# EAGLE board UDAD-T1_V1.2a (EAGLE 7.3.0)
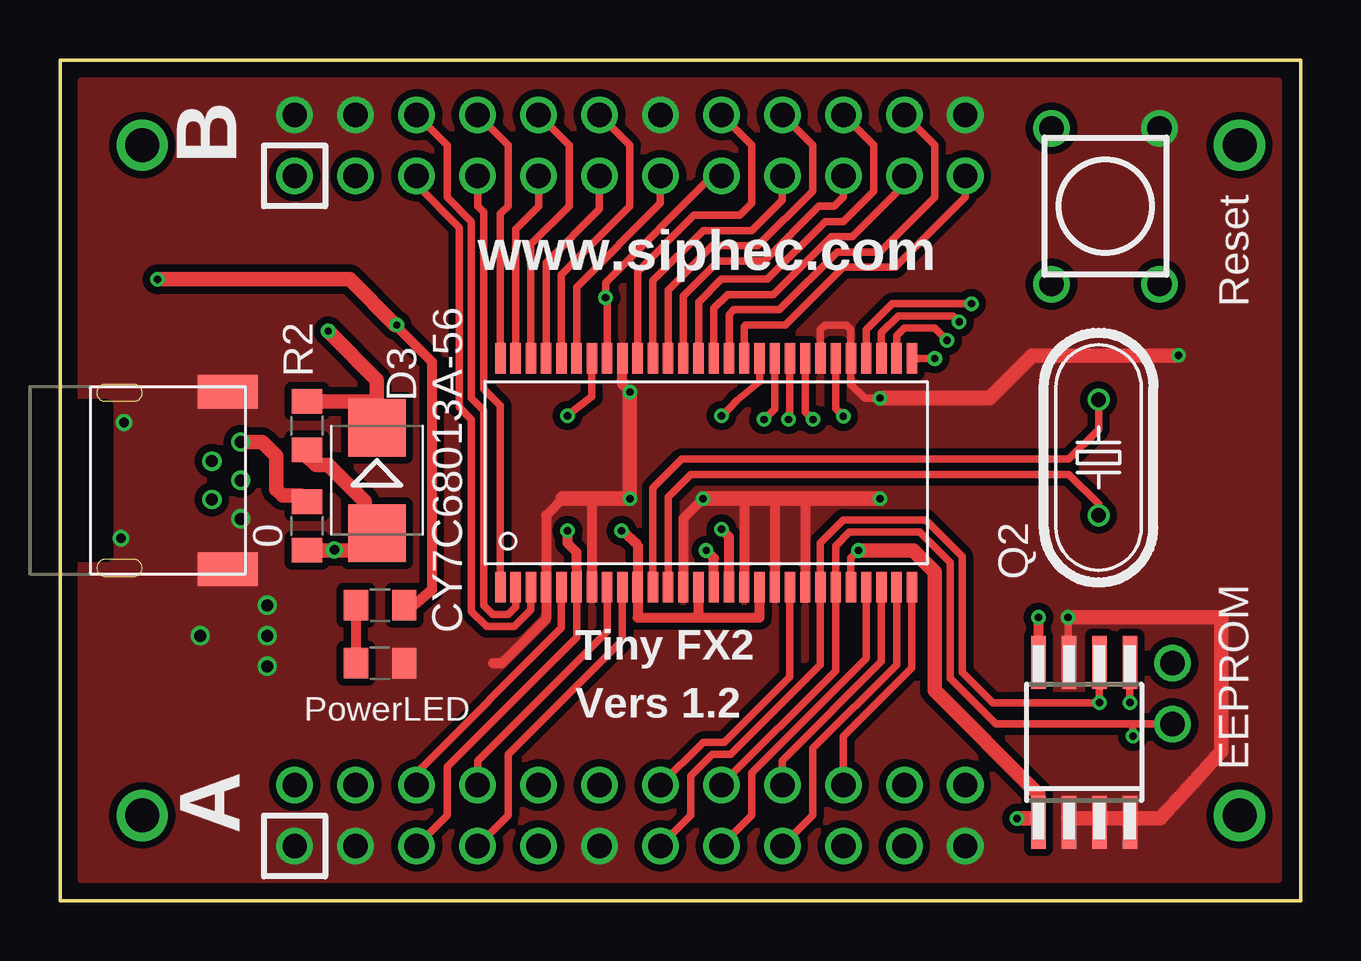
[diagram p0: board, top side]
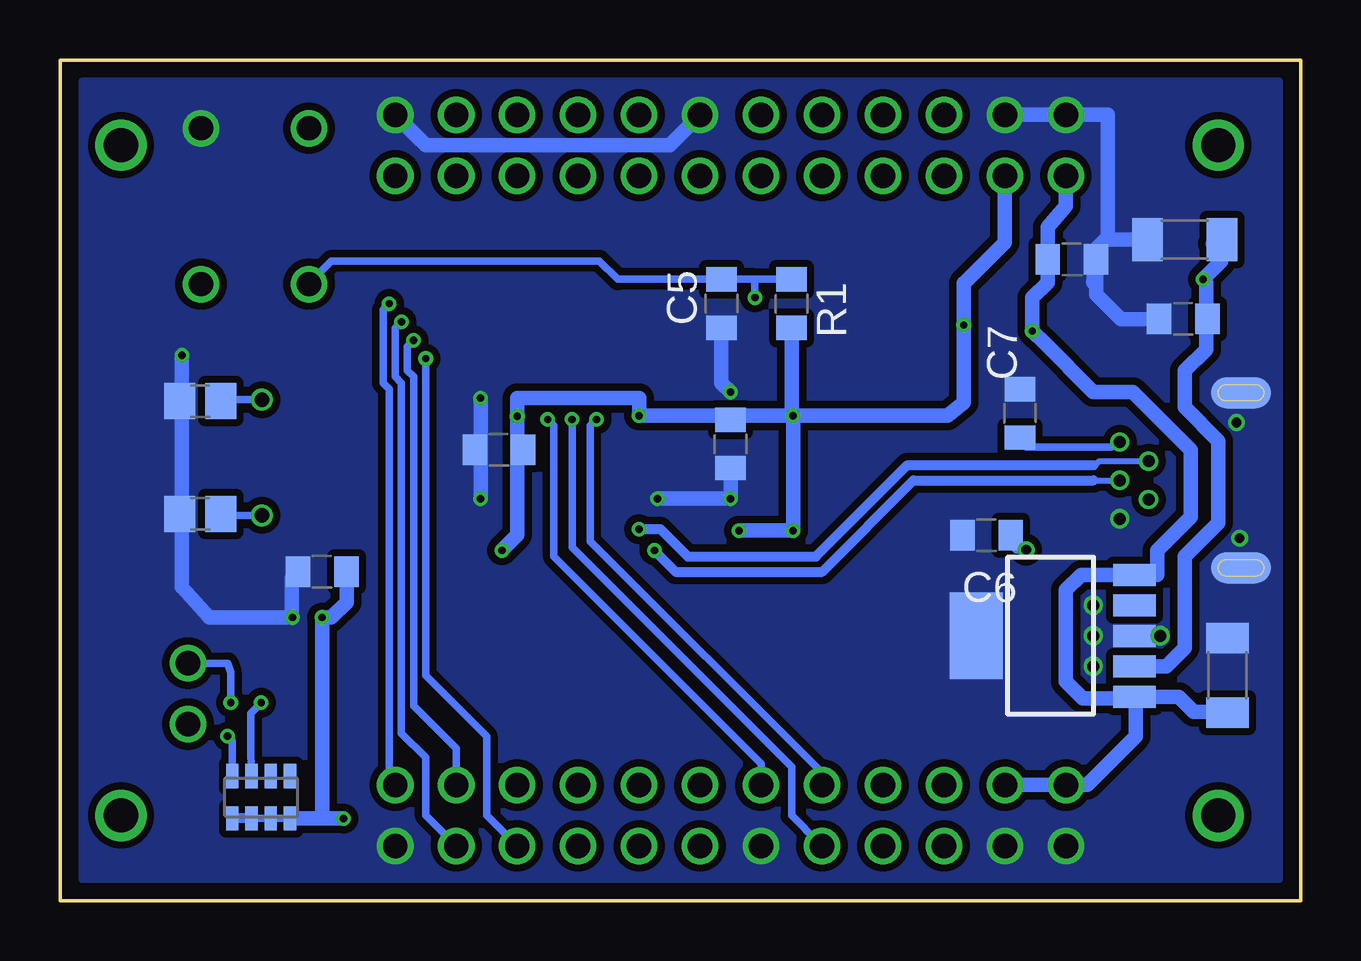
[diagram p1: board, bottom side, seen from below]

Size 51.69 x 35.05 mm. Coordinates in mm from the lower left corner, seen from the top.
Outline: 0,35.05 51.69,35.05 51.69,0 0,0 0,35.05
Copper layers (1*16): Top 0.035mm / dielectric 1.5mm / Bottom 0.035mm
Design rules "6mil Default": minimum track width 6mil, minimum drill 12mil, track to track 6mil, track to pad 6mil, pad to pad 6mil, via to via 6mil, smd to smd 0mil, copper to edge 6mil, drill to drill 6mil, minimum pad ring 6mil, minimum via ring 6mil, stop-mask expansion 2mil, vias tented up to drill 12.5mil, thermal gap 10mil

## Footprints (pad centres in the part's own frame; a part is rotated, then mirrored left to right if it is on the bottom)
C0805 = smd 1.016 x 1.27: 1 -1.009,0; 2 1.009,0
C1206 = smd 1.27 x 1.778: 1 -1.559,0; 2 1.559,0
C0805' = smd 1.3 x 1.5: 1 -0.85,0; 2 0.85,0
SMB = smd 2.4 x 2.4: A 2.2,0; C -2.2,0
PB_PHAP3301 = drill 1.016: 1 -3.25,2.25; 2 3.25,2.25; 3 -3.25,-2.25; 4 3.25,-2.25
MINI-USB-TH = drill 0.5: 1 8.8,1.6; 2 7.6,0.8; 3 8.8,0; 4 7.6,-0.8; 5 8.8,-1.6 | smd 2.5 x 1.4: S1 8.25,3.7; S2 8.25,-3.7 | smd 2.5 x 1.3 bottom: S3 3.75,3.65; S4 3.75,-3.65
JUMPER_1 = drill 1.016: P$1 0,-1.27; P$2 0,1.27
SO-08M = smd 0.6 x 2.2: 1 -1.905,-3.33; 2 -0.635,-3.33; 3 0.635,-3.33; 4 1.905,-3.33; 5 1.905,3.33; 6 0.635,3.33; 7 -0.635,3.33; 8 -1.905,3.33
SSOP56 = smd 1.27 x 0.432: 1 -4.763,8.572; 2 -4.763,7.938; 3 -4.763,7.303; 4 -4.763,6.668; 5 -4.763,6.032; 6 -4.763,5.397; 7 -4.763,4.763; 8 -4.763,4.128; 9 -4.763,3.493; 10 -4.763,2.857; 11 -4.763,2.223; 12 -4.763,1.587; 13 -4.763,0.953; 14 -4.763,0.318; 15 -4.763,-0.318; 16 -4.763,-0.953; 17 -4.763,-1.587; 18 -4.763,-2.223; 19 -4.763,-2.857; 20 -4.763,-3.493; 21 -4.763,-4.128; 22+ -4.763,-4.763; 23 -4.763,-5.397; 24 -4.763,-6.032; 25 -4.763,-6.668; 26 -4.763,-7.303; 27 -4.763,-7.938; 28 -4.763,-8.572; 29 4.763,-8.572; 30 4.763,-7.938; 31 4.763,-7.303; 32 4.763,-6.668; 33 4.763,-6.032; 34 4.763,-5.397; 35 4.763,-4.763; 36 4.763,-4.128; 37 4.763,-3.493; 38 4.763,-2.857; 39 4.763,-2.223; 40 4.763,-1.587; 41 4.763,-0.953; 42 4.763,-0.318; 43 4.763,0.318; 44 4.763,0.953; 45 4.763,1.587; 46 4.763,2.223; 47 4.763,2.857; 48 4.763,3.493; 49 4.763,4.128; 50 4.763,4.763; 51 4.763,5.397; 52 4.763,6.032; 53 4.763,6.668; 54 4.763,7.303; 55 4.763,7.938; 56 4.763,8.572
HC49U-V = drill 0.61: 1 -2.413,0; 2 2.413,0
SOT223-5 = smd 0.914 x 1.778: 1 -2.54,-3.493; 2 -1.27,-3.493; 3 0,-3.493; 4 1.27,-3.493; 5 2.54,-3.493 | smd 3.6 x 2.2: 6 0,3.099
R-4P = smd 0.508 x 1.016: 1 -1.2,-0.88; 2 -0.4,-0.88; 3 0.4,-0.88; 4 1.2,-0.88; 5 1.2,0.88; 6 0.4,0.88; 7 -0.4,0.88; 8 -1.2,0.88
MA12-2 = drill 1.016: 1 -13.97,-1.27; 2 -13.97,1.27; 3 -11.43,-1.27; 4 -11.43,1.27; 5 -8.89,-1.27; 6 -8.89,1.27; 7 -6.35,-1.27; 8 -6.35,1.27; 9 -3.81,-1.27; 10 -3.81,1.27; 11 -1.27,-1.27; 12 -1.27,1.27; 13 1.27,-1.27; 14 1.27,1.27; 15 3.81,-1.27; 16 3.81,1.27; 17 6.35,-1.27; 18 6.35,1.27; 19 8.89,-1.27; 20 8.89,1.27; 21 11.43,-1.27; 22 11.43,1.27; 23 13.97,-1.27; 24 13.97,1.27

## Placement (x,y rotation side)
0  [C0805]  10.29,15.62 90 top
C1  [C1206]  3.05,9.4 270 bottom
C2  [C1206]  4.83,27.56 180 bottom
C3  [C0805]  4.89,24.26 180 bottom
C4  [C0805]  9.52,26.73 180 bottom
C5  [C0805]  24.13,24.89 90 bottom
C6  [C0805]  13.08,15.24 180 bottom
C7  [C0805]  11.68,20.32 90 bottom
C8  [C0805']  45.85,20.83 180 bottom
C9  [C0805']  45.85,16.13 180 bottom
C10  [C0805]  40.77,13.72 180 bottom
C11  [C0805]  23.75,19.05 270 bottom
C12  [C0805]  33.4,18.8 180 bottom
D3  Schottky  [SMB]  13.21,17.53 270 top
E$1  [PB_PHAP3301]  43.56,28.96 90 top
E$3  [MINI-USB-TH]  -1.27,17.53 0 top
E$4  [JUMPER_1]  46.35,8.64 0 top
IC1  [SO-08M]  42.67,6.6 0 top
IC2  [SSOP56]  26.92,17.84 90 top
LED1  [C0805]  13.34,9.91 180 top
Q2  24 MHz  [HC49U-V]  43.28,18.48 90 top
R1  [C0805]  21.21,24.89 270 bottom
R2  [C0805]  10.29,19.81 270 top
R3  [C0805]  13.34,12.32 0 top
REG104  [SOT223-5]  10.41,11.05 90 bottom
RN1  [R-4P]  43.31,4.32 180 bottom
SV1  [MA12-2]  23.75,31.5 0 top
SV2  [MA12-2]  23.75,3.56 0 top

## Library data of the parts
0 C1-C7 C10-C12 LED1 R1-R3 = my_rcl
C8 C9 = rcl
D3 = diode
E$1 = SIP1
E$3 = Mini-USB-con
E$4 Q2 REG104 SV1 SV2 = my_lbr
IC1 = microchip
IC2 RN1 = FX2-56-TB

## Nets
3P3: C2.1 C3.1 C10.1 C11.1 C12.1 IC1.1 IC1.8 IC2.6 IC2.10 IC2.14 IC2.18 IC2.24 IC2.34 IC2.39 IC2.50 R1.2 R3.2 REG104.2 RN1.5 RN1.6 RN1.7 RN1.8 SV1.3 SV2.5
5P-USB: 0.2 C7.1 E$3.1
5V: C1.2 C4.2 D3.C R2.1 REG104.1 REG104.5 SV1.1 SV2.2 SV2.4
ADJ: REG104.4
CLKOUT: IC2.5 SV2.6
CTL0: IC2.36 SV2.12
CTL1: IC2.37 SV2.9
CTL2: IC2.38 SV2.10
D+: E$3.3 IC2.15
D-: E$3.2 IC2.16
GND: C1.1 C2.2 C3.2 C4.1 C5.1 C6.2 C7.2 C8.2 C9.2 C10.2 C11.2 C12.2 E$1.4 E$3.5 E$3.S1 E$3.S2 E$3.S3 E$3.S4 IC1.2 IC1.3 IC1.4 IC1.7 IC2.4 IC2.7 IC2.13 IC2.17 IC2.19 IC2.21 IC2.33 IC2.35 IC2.48 LED1.1 REG104.3 REG104.6 SV1.2 SV1.4 SV1.14 SV1.24 SV2.1 SV2.3 SV2.11 SV2.23
IFCLK: IC2.20 SV2.14
PA0: IC2.40 SV1.23
PA1: IC2.41 SV1.22
PA2: IC2.42 SV1.21
PA3: IC2.43 SV1.20
PA4: IC2.44 SV1.19
PA5: IC2.45 SV1.18
PA6: IC2.46 SV1.17
PA7: IC2.47 SV1.16
PB0: IC2.25 SV2.15
PB1: IC2.26 SV2.18
PB2: IC2.27 SV2.17
PB3: IC2.28 SV2.20
PB4: IC2.29 SV2.19
PB5: IC2.30 SV2.22
PB6: IC2.31 SV2.21
PB7: IC2.32 SV2.24
PD0: IC2.52 SV1.12
PD1: IC2.53 SV1.11
PD2: IC2.54 SV1.10
PD3: IC2.55 SV1.9
PD4: IC2.56 SV1.8
PD5: IC2.1 SV1.7
PD6: IC2.2 SV1.6
PD7: IC2.3 SV1.5
RDY0: IC2.8 SV2.8
RDY1: IC2.9 SV2.7
RESET: C5.2 E$1.1 IC2.49 R1.1 SV1.15
S$1: LED1.2 R3.1
S$6: 0.1 C6.1 D3.A R2.2
SCL: IC1.6 IC2.22+ RN1.3 SV2.13
SDA: E$4.P$1 IC2.23 RN1.4 SV2.16
SDA_JUMPER: E$4.P$2 IC1.5
WAKEUP: IC2.51 SV1.13
XTALIN: C9.1 IC2.12 Q2.1
XTALOUT: C8.1 IC2.11 Q2.2

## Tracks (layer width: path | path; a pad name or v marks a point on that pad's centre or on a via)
3P3  (via drill 0.3)
  Top 0.305: IC2.18 | IC2.14 | IC2.50 | 22.16,21.02 IC2.50 | 22.16,21.02 IC2.50 | IC2.39 29.15,21.65 28.19,20.86 27.57,20.18 | v21.14,20.23 22.16,21.02 | 27.57,20.18 v27.56,20.23 27.57,20.18 | IC2.24 | IC1.8 40.76,10.22 | v14.03,24 14.1,24 | IC2.34 32.32,20.51 v32.64,20.19 | IC2.24 32.96,14.29 v33.27,14.61 | IC2.6 21.53,10.99 16.13,5.59 16.13,3.56 SV2.5 | SV2.5 | IC2.10
  Top 0.406: IC2.6 21.51,14.54 21.14,14.91 v21.14,15.43 | v23.4,15.43 24.07,14.83 IC2.10 24.07,11.81 26.61,11.81 | 26.61,11.81 IC2.14 | IC2.18 29.15,11.81 26.61,11.81 | R3.2 14.73,12.32 15.49,12.95 15.49,22.48 13.97,24 | 36.45,8.89 36.45,8.76 | 40.77,4.44 40.77,3.43 | v40.77,11.81 IC1.8
  Top 0.61: v4.06,25.91 12.07,25.91 13.97,24 v14.03,24 | v33.27,14.61 35.56,14.61 36.45,13.72 36.45,8.89 | 40.77,3.43 IC1.1 | 40.77,3.43 40.77,3.68 | 36.45,8.76 40.77,4.44 | 40.77,3.43 v39.88,3.43
  Bottom 0.305: 14.03,25.75 14,25.75 | v23.4,15.43 23.3,15.43 | 21.37,20.23 21.14,20.19 | C3.1 3.88,24.19 3.94,24.13 3.81,24 | RN1.6 43.7,3.43 42.92,3.43 RN1.7 42.9,3.43 42.1,3.43 RN1.8 | C10.1 | SV1.3
  Bottom 0.406: C2.1 3.65,27.4 | RN1.6 RN1.5 | v39.88,3.43 40.77,3.43
  Bottom 0.61: SV1.3 12.32,27.43 14,25.75 | 14.03,25.75 v14.03,24 14.03,20.77 14.7,20.23 v21.14,20.23 | v21.14,20.23 21.37,20.23 | v23.4,15.43 v21.14,15.43 21.14,20.19 | 23.75,20.23 v21.14,20.23 | 23.75,20.23 v27.56,20.23 | v27.56,20.23 | 3.65,27.4 3.56,27.3 | v27.56,20.23 27.56,20.96 32.64,20.96 v32.64,20.19 32.64,18.8 | C11.1 23.75,20.23 | 32.64,18.8 32.64,15.24 v33.27,14.61 | 32.64,18.8 C12.1 | 21.14,20.19 21.08,20.19 | v21.14,20.23 21.14,20.19 | R1.2 21.21,20.19 21.14,20.19 | 40.77,3.43 v40.77,11.81 40.39,11.81 39.75,12.45 C10.1 | v39.88,3.43 42.1,3.43 | REG104.2 5.59,9.78 4.83,10.54 4.83,14.35 3.43,15.75 3.43,19.18 4.83,20.57 4.83,22.1 3.94,22.99 3.94,24.26 | 3.94,24.26 3.94,25.78 v4.06,25.91 3.3,26.67 3.3,27.56 C2.1 | 3.94,24.26 C3.1
5P-USB
  Top 0.61: E$3.1 8.43,19.13 9.02,18.54 9.02,17.14 9.27,16.89 10.03,16.89 0.2
  Bottom 0.305: C7.1 11.56,19.18 11.56,19.05 11.43,18.92 7.87,18.92 7.62,19.18 7.57,19.13 E$3.1
  Bottom 0.61: 7.49,19.18 arc-90 E$3.1
5V  (via drill 0.3)
  Top 0.61: 13.21,20.83 13.21,21.72 v11.18,23.75 | 13.21,20.83 D3.C | 13.21,20.83 13.08,20.83 13.07,20.82 R2.1
  Bottom 0.305: 9.78,30.07 9.78,30.1 SV1.1 | SV1.1
  Bottom 0.61: C1.2 3.27,7.84 3.3,7.87 4.45,7.87 5.08,8.51 6.6,8.51 | SV2.2 | SV2.2 SV2.4 | SV2.2 8.89,4.83 6.86,6.86 6.86,8.26 6.92,8.32 6.92,8.45 | 6.6,8.51 6.48,8.38 | 6.6,8.51 REG104.1 6.92,8.45 | 6.92,8.45 6.6,8.51 | 6.92,8.45 9.08,8.45 9.78,9.14 9.78,12.95 9.14,13.59 REG104.5 5.97,13.59 5.97,14.61 4.57,16 4.57,18.8 6.99,21.21 8.64,21.21 10.67,23.24 | 10.67,23.24 8.76,21.34 | 10.67,23.24 v11.18,23.75 11.18,25.15 10.54,25.78 C4.2 10.53,28.07 9.78,28.96 9.78,30.1
CLKOUT
  Top 0.305: IC2.5 20.89,11.37 14.86,5.33 14.86,4.95 | SV2.6 | 14.86,4.95 | 14.86,4.95 SV2.6
CTL0  (via drill 0.3)
  Top 0.305: IC2.36 31.05,20.38 v31.37,20.07
  Bottom 0.305: v31.37,20.07 31.12,19.81 31.12,14.35 22.48,5.71 SV2.12 | SV2.12
CTL1  (via drill 0.3)
  Top 0.305: IC2.37 30.42,20.13 v30.35,20.07
  Bottom 0.305: v30.35,20.07 30.35,14.73 21.21,5.59 21.21,3.56 20.07,2.41 | SV2.9 | 20.07,2.41 | 20.07,2.41 SV2.9
CTL2  (via drill 0.3)
  Top 0.305: IC2.38 29.78,20.51 v29.34,20.07
  Bottom 0.305: v29.34,20.07 29.59,19.81 29.59,14.99 19.94,5.33 SV2.10 | SV2.10
D+  (via drill 0.3)
  Top 0.406: IC2.15 27.24,14.29 v26.92,14.61
  Bottom 0.254: 8.64,17.53 E$3.3
  Bottom 0.406: v26.92,14.61 26.04,13.72 19.94,13.72 16.13,17.53 8.64,17.53
D-  (via drill 0.3)
  Top 0.406: IC2.16 27.88,15.18 v27.56,15.49
  Bottom 0.254: E$3.2 8.39,18.33 8.56,18.16 8.64,18.16
  Bottom 0.406: v27.56,15.49 26.67,15.49 25.53,14.35 20.19,14.35 16.38,18.16 8.64,18.16
GND  (via drill 0.3, 0.4, 0.5)
  Top 0.305: 44.58,2.54 IC1.4 44.49,3.4 43.27,3.4 IC1.3 43.22,3.4 42.01,3.4 IC1.2 | SV2.1 9.94,2.29 | 42.01,10 42.01,9.75 | 42.01,10 IC1.7 | v42.01,11.81 42.01,10 | IC2.35 31.69,23.81 31.88,24 32.77,24 32.96,23.81 IC2.33 | IC2.33 | IC2.33 32.96,21.53 33.53,20.96 v34.16,20.96 | IC2.7 22.16,13.4 | IC2.17
  Top 0.406: 18.03,9.91 18.41,9.91 20.26,11.75 IC2.4 20.26,16.07 20.95,16.76 | IC2.21 31.05,16.76 30.86,16.76 | IC2.19 29.78,16.76 30.1,16.76 | IC2.17 28.51,16.76 28.19,16.76 | IC2.7 22.16,16.76 22.73,16.76 | IC2.13 25.97,15.94 v26.8,16.76 | IC2.48 23.43,21.53 v23.75,21.21 | LED1.1 14.61,9.78
  Top 0.61: v46.61,22.73 40.51,22.73 38.73,20.96 v34.16,20.96 | v34.16,16.76 30.86,16.76 30.1,16.76 28.19,16.76 v26.8,16.76 | 20.95,16.76 22.73,16.76 v23.75,16.76 v23.75,21.21 | 42.01,3.4 42.01,3.43 45.85,3.43 47.24,4.95 48.39,6.22 48.39,11.81 v42.01,11.81
  Bottom 0.305: SV1.2 9.94,32.77 | SV1.2 | C10.2 42.04,13.46 | v42.01,11.81 41.91,11.81 42.04,11.94
  Bottom 0.61: SV1.4 SV1.2 8.03,32.77 8.03,27.56 | 8.03,27.56 C2.2 | SV1.14 | SV1.14 26.29,31.5 36.45,31.5 SV1.24 | SV1.24 | v42.01,11.81 45.47,11.81 46.61,13.08 46.61,16.13 | 46.61,16.13 C9.2 | 46.61,20.83 46.61,16.13 | 46.61,20.83 C8.2 | v46.61,22.73 46.61,20.83 | 34.16,18.8 v34.16,20.96 | 34.16,18.8 C12.2 | v34.16,16.76 34.16,18.8 | v26.8,16.76 v23.75,16.76 C11.2 | 8.03,27.56 8.13,27.56 8.51,27.18 8.51,25.78 | 8.51,25.78 8.51,25.27 7.49,24.26 C3.2 | 8.51,25.78 8.64,25.78 8.64,25.79 C4.1 | C5.1 24.13,21.59 v23.75,21.21 | 42.04,11.94 42.04,13.46
  other vias: 2.54,15.11 2.67,19.94 5.84,11.05 8.64,12.32 8.64,11.05 8.64,9.78
  pour Top (isolate 0.305, no thermals): 0.89,34.16 50.77,34.16 50.77,0.89 0.89,0.89
  pour Bottom (isolate 0.305, no thermals): 0.89,34.16 50.77,34.16 50.77,0.89 0.89,0.89
IFCLK
  Top 0.305: IC2.20 30.42,9.33 27.69,6.6 26.8,6.6 SV2.14 | SV2.14
  Bottom 0.305: SV2.14
PA0
  Top 0.305: SV1.23 | SV1.23 37.72,29.34 34.8,26.42 32.64,26.42 30.23,24 28.57,24 28.51,23.94 IC2.40
PA1
  Top 0.305: SV1.22 | SV1.22 36.45,31.5 36.45,29.34 34.16,27.05 32.38,27.05 29.97,24.64 28.07,24.64 27.88,24.45 IC2.41
  Bottom 0.305: SV1.22
PA2
  Top 0.305: IC2.42 27.24,24.7 27.81,25.27 29.72,25.27 32.13,27.69 33.02,27.69 35.18,29.85 | 35.18,29.85 | 35.18,29.85 SV1.21
PA3
  Top 0.305: IC2.43 26.61,24.96 27.56,25.91 29.46,25.91 31.88,28.32 32.64,28.32 33.91,29.59 33.91,31.5 SV1.20 | SV1.20
PA4
  Top 0.305: IC2.44 25.97,25.21 27.43,26.67 29.34,26.67 31.62,28.96 32.26,28.96 32.64,29.34 SV1.19 | 32.64,30.1 | SV1.19 32.64,30.1 | SV1.19
PA5
  Top 0.305: IC2.45 25.34,25.46 27.18,27.3 29.08,27.3 31.37,29.59 31.37,31.5 SV1.18 | SV1.18
PA6
  Top 0.305: IC2.46 24.7,25.84 26.8,27.94 28.83,27.94 30.1,29.21 30.1,30.1 | 30.1,30.1 | 30.1,30.1 SV1.17
PA7
  Top 0.305: IC2.47 24.07,26.23 26.42,28.57 28.32,28.57 28.83,29.08 28.83,31.5 SV1.16 | SV1.16
PB0
  Top 0.305: IC2.25 33.59,10.1 28.83,5.33 28.83,3.56 SV2.15 | SV2.15
PB1
  Top 0.305: IC2.26 34.23,9.97 30.1,5.84 SV2.18 | SV2.18
PB2
  Top 0.305: IC2.27 34.86,9.84 31.37,6.35 31.37,3.56 SV2.17 | SV2.17
PB3
  Top 0.305: IC2.28 35.5,9.71 32.64,6.86 SV2.20
PB4  (via drill 0.3)
  Top 0.305: v36.45,22.61 IC2.29 | v36.45,22.61
  Bottom 0.305: v36.45,22.61 36.45,9.4 33.91,6.86 33.91,3.56 SV2.19 | SV2.19
PB5  (via drill 0.3)
  Top 0.305: IC2.30 34.86,23.56 35.18,23.88 36.45,23.88 v36.96,23.37
  Bottom 0.305: v36.96,23.37 37.21,23.11 37.21,22.1 36.96,21.84 36.96,8.13 35.18,6.35 SV2.22 | SV2.22 | SV2.22
PB6  (via drill 0.3)
  Top 0.305: IC2.31 34.23,23.69 34.92,24.38 37.21,24.38 v37.46,24.13
  Bottom 0.305: v37.46,24.13 37.72,23.88 37.72,21.84 37.46,21.59 37.46,6.98 36.45,5.97 36.45,3.56 SV2.21 | SV2.21
PB7  (via drill 0.3)
  Top 0.305: IC2.32 33.59,23.81 34.67,24.89 v37.97,24.89
  Bottom 0.305: v37.97,24.89 38.23,24.64 38.23,21.59 37.97,21.34 37.97,5.08 SV2.24 | SV2.24
PD0
  Top 0.305: IC2.52 20.89,26.1 23.75,28.96 23.75,31.5 SV1.12 | SV1.12
PD1
  Top 0.305: IC2.53 20.26,26.61 22.48,28.83 SV1.11 | SV1.11
PD2
  Top 0.305: IC2.54 19.62,27.37 21.21,28.96 21.21,31.5 SV1.10 | SV1.10
PD3
  Top 0.305: IC2.55 18.99,28 19.94,28.96 19.94,30.1 | 19.94,30.1 | 19.94,30.1 SV1.9
PD4
  Top 0.305: IC2.56 18.35,28.64 18.67,28.96 18.67,31.5 SV1.8 | SV1.8
PD5
  Top 0.305: IC2.1 18.35,20.64 17.65,21.34 17.65,28.7 17.4,28.96 SV1.7 | SV1.7
PD6
  Top 0.305: IC2.2 18.99,12.26 18.67,11.94 18.03,11.94 17.65,12.32 17.65,20.45 17.14,20.96 17.14,28.32 16.13,29.34 16.13,31.5 SV1.6 | SV1.6
PD7
  Top 0.305: IC2.3 19.62,12.13 18.92,11.43 17.78,11.43 17.14,12.07 17.14,20.07 16.64,20.57 16.64,28.07 14.86,29.85 SV1.5
RDY0
  Top 0.305: IC2.8 22.8,11.24 17.4,5.84 SV2.8 | SV2.8
RDY1
  Top 0.305: IC2.9 23.43,10.86 18.67,6.1 18.67,3.56 SV2.7 | SV2.7
RESET  (via drill 0.3)
  Top 0.305: IC2.49 22.8,22.45 | IC2.49 | IC2.49 | IC2.49 | IC2.49 | IC2.49 22.8,25.08 v22.73,25.15 22.73,25.78 27.18,30.23 SV1.15
  Bottom 0.305: R1.1 22.73,25.91 | v22.73,25.15 22.73,25.91 | 22.73,25.91 C5.2 | C5.2 | C5.2 28.45,25.91 29.21,26.67 40.39,26.67 41.35,25.71 | 41.35,25.71 41.4,25.65 | 41.35,25.71 E$1.1
S$1
  Top 0.406: R3.1 12.32,10.41 LED1.2
S$2  (via drill 1.42)
  other vias: 49.15,31.5
S$3  (via drill 1.42)
  other vias: 3.43,3.56
S$4  (via drill 1.42)
  other vias: 3.43,31.5
S$5  (via drill 1.42)
  other vias: 49.15,3.56
S$6  (via drill 0.4)
  Top 0.305: v11.43,14.63 11.43,14.61
  Top 0.61: 0.1 11.43,14.61 12.58,14.61 13.21,15.24 D3.A 12.83,15.37 12.7,15.49 12.7,16.64 11.18,18.16 10.67,18.16 10.29,18.54 R2.2 10.54,18.54
  Bottom 0.305: C6.1 12.07,14.87 11.84,14.63 v11.43,14.63
SCL  (via drill 0.3)
  Top 0.305: SV2.13 | SV2.13 26.29,3.56 26.29,5.21 27.18,6.1 27.94,6.1 31.69,9.84 IC2.22+ 31.69,14.92 32.64,15.88 36.07,15.88 37.59,14.35 37.59,9.53 38.86,8.26 40.01,8.26 | IC1.6 v43.31,8.26 40.01,8.26 | 40.01,8.26 39.88,8.26
  Bottom 0.305: RN1.3 43.75,6.1 43.75,7.81 v43.31,8.26
SDA  (via drill 0.3)
  Top 0.305: SV2.16 | SV2.16 32.32,9.59 IC2.23 32.32,14.79 32.89,15.37 35.81,15.37 37.08,14.1 37.08,9.27 38.99,7.37 44.7,7.37 | 44.7,7.37 v44.7,6.86 | 44.7,7.37 E$4.P$1
  Bottom 0.305: RN1.4 44.51,6.66 v44.7,6.86
SDA_JUMPER  (via drill 0.3)
  Top 0.305: v44.58,8.26 IC1.5
  Bottom 0.305: E$4.P$2 44.7,9.91 44.58,9.53 v44.58,8.26
WAKEUP
  Top 0.305: SV1.13 | IC2.51 21.53,25.59 25.02,29.08 25.02,30.1 | 25.02,30.1 | 25.02,30.1 SV1.13
XTALIN
  Top 0.305: Q2.1 43.27,16.54 42.04,17.78 26.29,17.78 25.34,16.83 IC2.12
  Bottom 0.305: C9.1 44.86,16.1 44.83,16.13 44.77,16.07 44.7,16.07 | Q2.1 44.7,16.07 | 44.7,16.07 44.7,16.13
XTALOUT
  Top 0.305: IC2.11 24.7,13.4 24.7,17.21 25.91,18.41 42.04,18.41 43.27,19.65 Q2.2
  Bottom 0.305: 44.96,20.83 44.96,20.84 C8.1 44.96,20.86 44.96,20.83 | 44.96,20.83 44.89,20.89 | Q2.2 44.96,20.89 44.96,20.83

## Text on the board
tPlace: B | www.siphec.com | Reset | CY7C68013A-56 | Tiny FX2 | Vers 1.2 | PowerLED | EEPROM | A
Measures: 0.685 | 17.4 | 0 | -0.685 | -17.4 | 0 | 1 | -0.55 | -14 | -0.935 | -19 | 25.4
